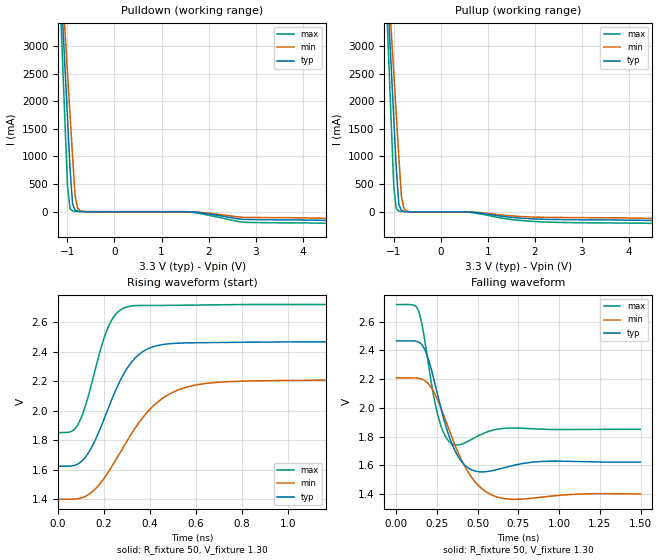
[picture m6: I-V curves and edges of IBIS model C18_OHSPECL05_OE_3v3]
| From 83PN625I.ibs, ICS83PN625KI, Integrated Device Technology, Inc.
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[Model] C18_OHSPECL05_OE_3v3
Model_type   Output_ECL
Polarity   Non-Inverting
|   typ   min   max
C_comp   2pF   1.5pF   2.5pF
Vmeas = 2.11V
Rref = 50
Cref = 0
Vref = 1.3V
|   typ   min   max
[Voltage range]   3.3V   3.135V   3.465V
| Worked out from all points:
|   rising waveform, R_fixture 50, V_fixture 1.30: 20-80 % time 146ps typ, 215ps min, 95ps max; typ from 1.62 V to 2.47 V
|   falling waveform, R_fixture 50, V_fixture 1.30: 20-80 % time 119ps typ, 179ps min, 76.1ps max; typ from 2.47 V to 1.62 V
[Pulldown]
|Voltage   I (typ)   I (min)   I (max)
-3.3V     49.22A     42.86A     60.01A
-1.46V    9.496A     9.003A     10.43A
-1V       1.719A     2.53A      485.2mA
-945mV    790.7mA    1.758A     52.22mA
-891mV    138.5mA    999.2mA    14.05mA
-837mV    26.96mA    288.2mA    7.503mA
-783mV    7.874mA    61.39mA    5.048mA
-674.9mV  1.518mA    4.525mA    1.866mA
1.54V     -841.1uA   -283.3uA   -2.691mA
2.728V    -137.9mA   -101.6mA   -188.6mA
4.866V    -169.3mA   -131.3mA   -220.8mA
6.6V      -240.4mA   -180.9mA   -324.4mA
[Pullup]
|Voltage   I (typ)   I (min)   I (max)
-3.3V     49.22A     42.86A     60.01A
-1.46V    9.496A     9.003A     10.43A
-1V       1.719A     2.53A      485.2mA
-945mV    790.7mA    1.758A     52.22mA
-891mV    138.5mA    999.2mA    14.05mA
-837mV    26.96mA    288.2mA    7.503mA
-783mV    7.874mA    61.38mA    5.048mA
-674.9mV  1.518mA    4.525mA    1.866mA
567.3mV   -2.281mA   -816.2uA   -5.352mA
2.08V     -131.5mA   -97.47mA   -178.8mA
4.866V    -169.2mA   -131.5mA   -220.5mA
6.6V      -239.5mA   -180.7mA   -322mA
[Ramp]
|   typ   min   max
dV/dt_r   0.673/0.223n   0.647/0.334n   0.693/0.143n
dV/dt_f   0.729/0.202n   0.676/0.291n   0.782/0.136n
R_load =   50.0000
[Rising Waveform]
R_fixture = 50
V_fixture = 1.30   | VCC_typ - 2V
V_fixture_max = 1.465   | VCC_max - 2V
V_fixture_min = 1.135   | VCC_min - 2V
C_fixture = 0.0p
| Time   typ   min   max
0s        1.623V     1.399V     1.851V
73.57ps   1.63V      1.401V     1.878V
124.6ps   1.697V     1.424V     2.061V
214.7ps   2.001V     1.574V     2.554V
249.2ps   2.133V     1.662V     2.65V
292.8ps   2.268V     1.777V     2.699V
352.9ps   2.382V     1.922V     2.712V
424.9ps   2.438V     2.047V     2.712V
579.6ps   2.459V     2.167V     2.715V
1.498ns   2.466V     2.208V     2.718V
[Falling Waveform]
R_fixture = 50
V_fixture = 1.30   | VCC_typ - 2V
V_fixture_max = 1.465   | VCC_max - 2V
V_fixture_min = 1.135   | VCC_min - 2V
C_fixture = 0.0p
| Time   typ   min   max
0s        2.466V     2.208V     2.718V
135.1ps   2.458V     2.205V     2.675V
187.7ps   2.368V     2.177V     2.368V
253.8ps   2.086V     2.053V     1.951V
295.8ps   1.901V     1.931V     1.813V
343.8ps   1.741V     1.785V     1.748V
453.5ps   1.573V     1.529V     1.775V
620.1ps   1.571V     1.379V     1.851V
893.4ps   1.627V     1.378V     1.851V
1.498ns   1.622V     1.4V       1.85V
